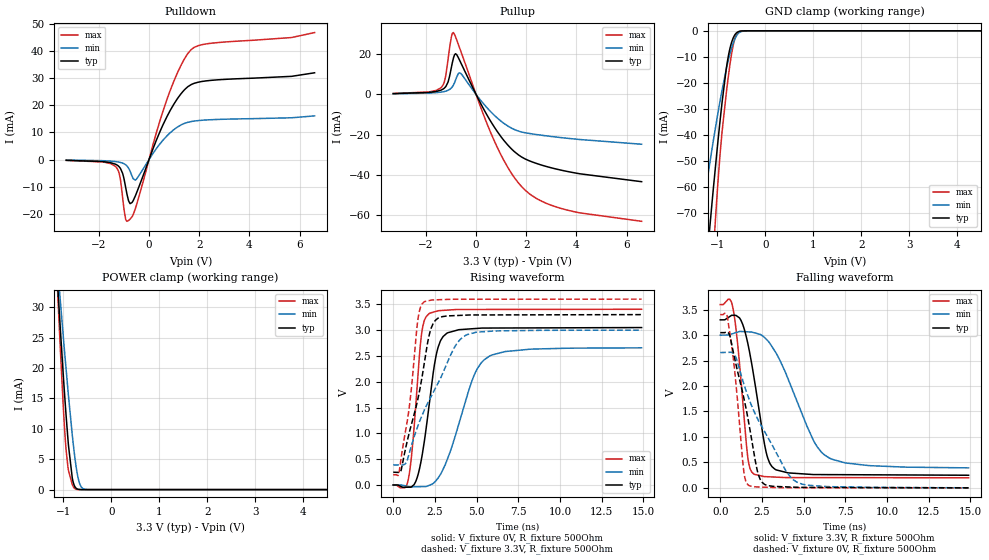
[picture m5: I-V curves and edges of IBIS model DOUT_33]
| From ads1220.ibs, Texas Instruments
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|   DOUT_33 Model
[Model]   DOUT_33
Model_type   3-state
Polarity   Non-Inverting
Vmeas = 1.65
Vref = 1.65
Cref = 15pF
Rref = 500
|   typ   min   max
|   (nom PVT)   (Fast PVT)   (slow PVT)
C_comp   2.929p   2.440p   3.431p
|C_comp (ON state)   3.054p   2.556p   3.558p
|C_comp (OFF state)   2.929p   2.440p   3.431p
| Where   nom PVT is  Nominal Process, 3.3V, 27C
|   Fast PVT is Strong Process, 3.6V, -40C
|   Slow PVT is Weak Process, 3.0V, 125C
[Voltage Range]   3.3   3   3.6
[Temperature Range]   27   125   -40
[Pullup Reference]   3.3   3   3.6
[Pulldown Reference]   0   0   0
[Power Clamp Reference]   3.3   3   3.6
[GND Clamp Reference]   0   0   0
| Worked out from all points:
|   slope of the pulldown table from 0 to 0.495 V, typ, clamps not added: 42.9 ohm
|   slope of the pullup table from 0 to 0.495 V, typ, clamps not added: 42.9 ohm
|   GND clamp passes 1 mA (typ) near -0.61 V on its own axis
|   POWER clamp passes 1 mA (typ) near -0.79 V on its own axis
|   falling waveform, V_fixture 3.3V, R_fixture 500Ohm: 20-80 % time 910ps typ, 2ns min, 548ps max; typ from 3.3 V to 0.248 V
|   rising waveform, V_fixture 0V, R_fixture 500Ohm: 20-80 % time 781ps typ, 1.57ns min, 497ps max; typ from 0 V to 3.05 V
|   rising waveform, V_fixture 3.3V, R_fixture 500Ohm: 20-80 % time 1.18ns typ, 2.15ns min, 735ps max; typ from 0.248 V to 3.3 V
|   falling waveform, V_fixture 0V, R_fixture 500Ohm: 20-80 % time 1.13ns typ, 2.28ns min, 590ps max; typ from 3.05 V to 0 V
[Pulldown]
|   Voltage   I(typ)   I(min)   I(max)
-3.3V     -288.8uA   -187.2uA   -310.5uA
-1.33V    -1.758mA   -765.4uA   -2.619mA
-1.181V   -2.776mA   -994.6uA   -5.449mA
-993.3mV  -7.307mA   -1.58mA    -18.7mA
-874.5mV  -13.02mA   -2.421mA   -22.81mA
-755.7mV  -16.29mA   -4.279mA   -22.03mA
-537.9mV  -13.25mA   -7.549mA   -17.94mA
709.5mV   15.75mA    8.689mA    22.07mA
1.264V    24.15mA    12.72mA    34.59mA
1.68V     27.68mA    14.03mA    40.59mA
2.373V    29.15mA    14.66mA    42.83mA
6.6V      32.04mA    16.12mA    46.89mA
[GND Clamp]
|   Voltage   I(typ)   I(min)   I(max)
-3.3V     -573.2mA   -376mA     -790.9mA
-1.488V   -145.8mA   -92.85mA   -208.7mA
-1.31V    -106.9mA   -69.41mA   -152.8mA
-1.221V   -88.11mA   -58.27mA   -125.3mA
-1.112V   -65.97mA   -45.27mA   -92.62mA
-1.092V   -62.06mA   -42.99mA   -86.84mA
-1.003V   -45.06mA   -33.08mA   -61.93mA
-904.2mV  -27.7mA    -22.89mA   -39.04mA
-795.3mV  -12.2mA    -13.14mA   -20.96mA
-666.6mV  -2.6mA     -4.574mA   -5.217mA
-557.7mV  -290.1uA   -882.3uA   -494.1uA
6.6V      0A         0A         0A
[Pullup]
|   Voltage   I(typ)   I(min)   I(max)
-3.3V     365.8uA    268.1uA    421.3uA
-1.389V   2.126mA    1.115mA    3.371mA
-1.261V   3.119mA    1.414mA    6.302mA
-1.122V   5.919mA    1.973mA    16.72mA
-983.4mV  13.32mA    3.162mA    28.43mA
-904.2mV  17.84mA    4.541mA    30.73mA
-815.1mV  20.2mA     7.121mA    28.52mA
-617.1mV  15.97mA    10.53mA    21.79mA
709.5mV   -15.91mA   -10.19mA   -22.63mA
1.957V    -32.13mA   -19.11mA   -47.65mA
3.482V    -37.95mA   -21.64mA   -57.06mA
6.6V      -43.45mA   -24.82mA   -63.15mA
[POWER Clamp]
|   Voltage   I(typ)   I(min)   I(max)
-3.3V     357.2mA    284.9mA    449.7mA
-1.112V   32.73mA    35.76mA    31.18mA
-1.102V   31.42mA    34.78mA    29.49mA
-1.063V   26.26mA    30.91mA    22.88mA
-993.3mV  17.74mA    24.34mA    12.34mA
-943.8mV  12.19mA    19.81mA    6.505mA
-894.3mV  7.278mA    15.44mA    3.136mA
-815.1mV  1.906mA    9.008mA    837.5uA
-745.8mV  317.1uA    4.371mA    91.31uA
-646.8mV  11.41uA    717.5uA    1.805uA
-498.3mV  48.78nA    12.41uA    0A
6.6V      0A         0A         0A
[Ramp]
R_load = 500
|   typ   min   max
dV/dt_r   1.82949/7.78901e-10   1.59388/1.56192e-09   2.04213/4.95395e-10
dV/dt_f   1.83121/9.0987e-10   1.56447/2.00297e-09   2.04137/5.4787e-10
[Falling Waveform]
V_fixture = 3.3V
V_fixture_min = 3V
V_fixture_max = 3.6V
R_fixture = 500Ohm
C_fixture = 0F
|   Time   V(typ)   V(min)   V(max)
0s        3.3V       3V         3.6V
764.6ps   3.389V     3.031V     3.527V
1.092ns   3.354V     3.065V     2.669V
1.647ns   2.847V     3.064V     614.4mV
2.007ns   2.202V     3.05V      273.7mV
2.768ns   682mV      2.918V     219.7mV
3.356ns   353.1mV    2.646V     210.6mV
5.578ns   261.4mV    941.5mV    201.5mV
6.542ns   260mV      586.5mV    201.1mV
14.9ns    248mV      392.6mV    197.7mV
[Rising Waveform]
V_fixture = 0V
V_fixture_min = 0V
V_fixture_max = 0V
R_fixture = 500Ohm
C_fixture = 0F
|   Time   V(typ)   V(min)   V(max)
0s        3.316nV    5.881nV    2.676nV
909.2ps   -43.18mV   -29.87mV   117.2mV
1.187ns   -10.48mV   -36.18mV   868.8mV
1.677ns   473.6mV    -31.77mV   2.868V
2.138ns   1.509V     -9.151mV   3.316V
2.568ns   2.503V     86.35mV    3.363V
2.988ns   2.874V     304.3mV    3.382V
4.823ns   3.028V     2.102V     3.4V
5.769ns   3.04V      2.495V     3.4V
14.9ns    3.049V     2.656V     3.404V
[Rising Waveform]
V_fixture = 3.3V
V_fixture_min = 3V
V_fixture_max = 3.6V
R_fixture = 500Ohm
C_fixture = 0F
|   Time   V(typ)   V(min)   V(max)
0s        247.9mV    388.3mV    197.7mV
341.7ps   242.7mV    388.1mV    221.9mV
985.5ps   1.044V     641.2mV    1.57V
1.487ns   1.68V      1.149V     3.221V
1.85ns    2.333V     1.438V     3.546V
2.184ns   2.937V     1.658V     3.574V
2.522ns   3.187V     1.87V      3.586V
3.676ns   3.28V      2.669V     3.597V
4.431ns   3.291V     2.912V     3.598V
14.9ns    3.3V       3V         3.6V
[Falling Waveform]
|Gnd
V_fixture = 0V
V_fixture_min = 0V
V_fixture_max = 0V
R_fixture = 500Ohm
C_fixture = 0F
|   Time   V(typ)   V(min)   V(max)
0s        3.049V     2.657V     3.404V
432.6ps   3.06V      2.661V     3.349V
865.9ps   2.54V      2.607V     2.301V
1.407ns   1.778V     2.053V     341.8mV
1.693ns   1.306V     1.777V     51.55mV
2.205ns   364mV      1.379V     17.81mV
2.501ns   113.1mV    1.197V     14.69mV
3.964ns   19.48mV    321.2mV    3.44mV
4.686ns   10.56mV    99.55mV    3.213mV
14.9ns    41.85uV    1.457mV    31.64nV
